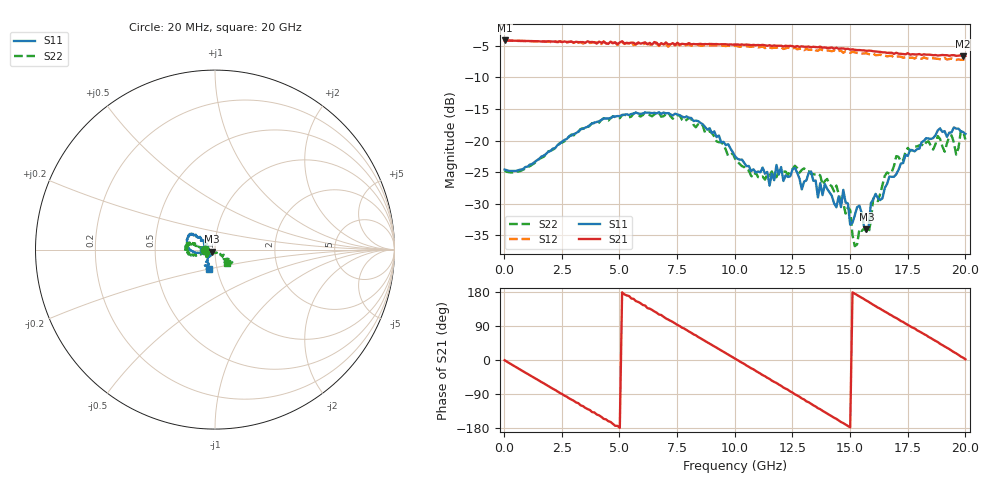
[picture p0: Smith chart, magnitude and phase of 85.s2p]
!Agilent Technologies,N5230A,US43500223,A.07.50.48
!Agilent N5230A: A.07.50.48
!Date: Wednesday, October 07, 2015 17:31:51
!Correction: S11(Full 2 Port(1,2))
!S21(Full 2 Port(1,2))
!S12(Full 2 Port(1,2))
!S22(Full 2 Port(1,2))
!S2P File: Measurements: S11, S21, S12, S22:
# Hz S  dB  R 50
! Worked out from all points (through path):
!   201 points, 20 MHz to 20 GHz, reference 50 ohm
!   highest |S21| = -4.13 dB at 20 MHz (marker M1); lowest = -6.6 dB at 19.9 GHz (marker M2)
!   group delay of S21, straight-line fit = 99.6 ps
!   lowest |S11| = -34.0 dB at 15.7 GHz (marker M3), VSWR 1.04, Z = 48.4 - j1.08 ohm
!   |S11| at or under -10 dB: start of sweep to end of sweep
!   |S22| runs from -36.7 to -15.5 dB; largest |S21 - S12| = 0.053
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2e7  -24.58 179.5  -4.13 -0.7  -4.13 -0.8  -24.80 -179.1
1.9181e9  -21.75 -166.4  -4.26 -69.0  -4.30 -69.9  -21.70 -162.6
3.4166e9  -18.13 -175.4  -4.39 -121.7  -4.61 -122.8  -18.05 -164.3
5.1149e9  -15.92 168.4  -4.26 178.5  -4.40 176.8  -15.98 -178.4
6.7133e9  -15.51 152.6  -4.90 120.0  -5.01 118.6  -15.63 176.0
8.012e9  -16.37 145.3  -4.55 75.2  -4.77 73.0  -16.42 165.9
1.001e10  -22.45 145.3  -4.76 3.6  -4.95 1.4  -22.86 176.9
1.15085e10  -27.12 152.0  -4.88 -50.0  -5.25 -53.1  -25.54 -150.4
1.2008e10  -24.19 166.3  -4.96 -68.0  -5.17 -71.1  -24.82 -143.2
1.34066e10  -26.36 178.9  -5.13 -119.5  -5.42 -121.8  -25.31 -148.9
1.44056e10  -30.56 -163.1  -5.29 -155.3  -5.94 -158.4  -27.12 -151.5
1.47053e10  -27.80 -157.7  -5.40 -166.5  -6.08 -169.3  -29.86 -148.4
1.5005e10  -33.32 -146.8  -5.58 -177.6  -6.10 179.2  -31.02 -127.9
1.52048e10  -31.82 -128.7  -5.61 175.0  -6.02 171.9  -36.72 -112.9
1.57043e10  -34.03 -145.9  -5.77 156.8  -6.16 153.5  -34.39 -60.8
1.59041e10  -29.87 -135.3  -5.76 149.5  -6.35 147.3  -32.67 -62.4
1.67033e10  -25.69 -132.6  -6.09 120.7  -6.58 118.9  -25.25 -35.9
1.82018e10  -20.01 -115.7  -6.33 68.5  -6.80 66.3  -20.87 -49.6
1.94006e10  -18.68 -104.5  -6.47 24.7  -6.99 21.2  -19.17 -45.8
1.96004e10  -18.10 -106.3  -6.57 17.4  -7.22 14.9  -22.22 -43.1
1.99001e10  -18.63 -103.7  -6.63 6.2  -7.18 3.2  -18.51 -40.0
2e10  -18.94 -106.1  -6.58 1.9  -7.13 -2.1  -19.83 -47.8
